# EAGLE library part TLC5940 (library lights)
16-channel LED Driver with Dot Correction and Grayscale PWM Control The TLC5940 is a 16-channel, constant-current sink LED driver. Each channel has an individually adjustable 4096-step grayscale PWM brightness control and a 64-step, constant-current sink (dot correction). The dot correction adjusts the brightness variations between LED channels and other LED drivers. The dot correction data is stored in an integrated EEPROM. Both grayscale control and dot correction are accessible via a serial interface. A single external resistor sets the maximum current value of all 16 channels. Packages: 28-pin HTSSOP 32-pin 5x5mm QFN 28-pin DIP
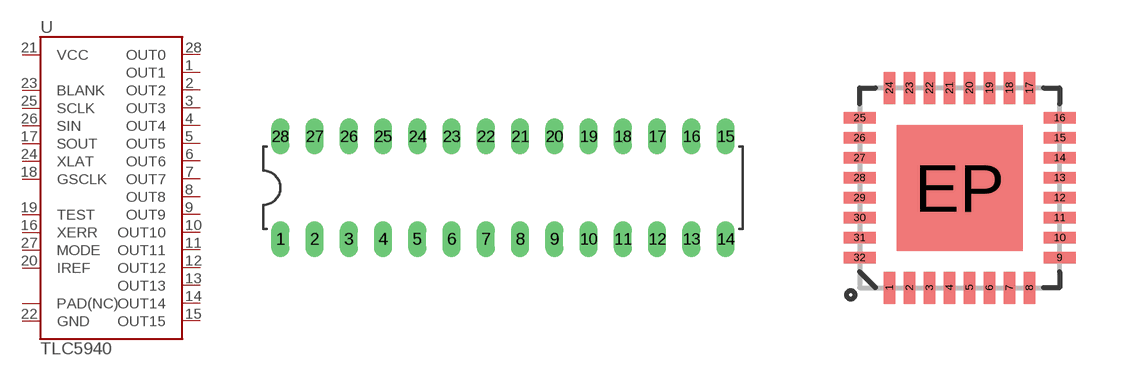
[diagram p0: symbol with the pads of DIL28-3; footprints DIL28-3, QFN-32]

Designator prefix U

## TLC5940-NT  [DIL28-3]
1  OUT1
2  OUT2
3  OUT3
4  OUT4
5  OUT5
6  OUT6
7  OUT7
8  OUT8
9  OUT9
10  OUT10
11  OUT11
12  OUT12
13  OUT13
14  OUT14
15  OUT15
16  XERR
17  SOUT
18  GSCLK
19  TEST
20  IREF
21  VCC
22  GND
23  BLANK
24  XLAT
25  SCLK
26  SIN
27  MODE
28  OUT0

## TLC5940-RHB (PROD_ID: IC-10398)  [QFN-32]
1  SCLK
2  SIN
3  MODE
4  OUT0
5  OUT1
6  OUT2
7  OUT3
8  OUT4
9  OUT5
10  OUT6
11  OUT7
14  OUT8
15  OUT9
16  OUT10
17  OUT11
18  OUT12
19  OUT13
20  OUT14
21  OUT15
22  XERR
23  SOUT
24  GSCLK
25  TEST
26  IREF
27  VCC
30  GND
31  BLANK
32  XLAT
EP  PAD(NC)

## TLC5940PWP  [TSSOP28-GROUNDPAD]
1  GND
2  BLANK
3  XLAT
4  SCLK
5  SIN
6  MODE
7  OUT0
8  OUT1
9  OUT2
10  OUT3
11  OUT4
12  OUT5
13  OUT6
14  OUT7
15  OUT8
16  OUT9
17  OUT10
18  OUT11
19  OUT12
20  OUT13
21  OUT14
22  OUT15
23  XERR
24  SOUT
25  GSCLK
26  TEST
27  IREF
28  VCC
29  PAD(NC)

## Footprint DIL28-3 (pad centres in mm)
Standard 28-pin DIP package. IC needs to have legs bent before insertion.
drill 0.813 long: 1 -16.51,-3.81; 2 -13.97,-3.81; 3 -11.43,-3.81; 4 -8.89,-3.81; 5 -6.35,-3.81; 6 -3.81,-3.81; 7 -1.27,-3.81; 8 1.27,-3.81; 9 3.81,-3.81; 10 6.35,-3.81; 11 8.89,-3.81; 12 11.43,-3.81; 13 13.97,-3.81; 14 16.51,-3.81; 15 16.51,3.81; 16 13.97,3.81; 17 11.43,3.81; 18 8.89,3.81; 19 6.35,3.81; 20 3.81,3.81; 21 1.27,3.81; 22 -1.27,3.81; 23 -3.81,3.81; 24 -6.35,3.81; 25 -8.89,3.81; 26 -11.43,3.81; 27 -13.97,3.81; 28 -16.51,3.81

## Footprint QFN-32 (pad centres in mm)
QFN 32-Pin package w/ Thermal Pad ***Unproven*** Applicable Parts: TLC5940
smd 0.285 x 0.8: 1 -1.75,-2.5; 2 -1.25,-2.5; 3 -0.75,-2.5; 4 -0.25,-2.5; 5 0.25,-2.5; 6 0.75,-2.5; 7 1.25,-2.5; 8 1.75,-2.5; 17 1.75,2.5; 18 1.25,2.5; 19 0.75,2.5; 20 0.25,2.5; 21 -0.25,2.5; 22 -0.75,2.5; 23 -1.25,2.5; 24 -1.75,2.5
smd 0.8 x 0.285: 9 2.5,-1.75; 10 2.5,-1.25; 11 2.5,-0.75; 12 2.5,-0.25; 13 2.5,0.25; 14 2.5,0.75; 15 2.5,1.25; 16 2.5,1.75; 25 -2.5,1.75; 26 -2.5,1.25; 27 -2.5,0.75; 28 -2.5,0.25; 29 -2.5,-0.25; 30 -2.5,-0.75; 31 -2.5,-1.25; 32 -2.5,-1.75
smd 3.15 x 3.15: EP 0,0

## Footprint TSSOP28-GROUNDPAD (pad centres in mm)
smd 0.8 x 0.25: 1 -2.921,4.298; 2 -2.921,3.637; 3 -2.921,2.977; 4 -2.921,2.317; 5 -2.921,1.656; 6 -2.921,0.996; 7 -2.921,0.335; 8 -2.927,-0.325; 9 -2.921,-0.985; 10 -2.921,-1.646; 11 -2.921,-2.306; 12 -2.921,-2.967; 13 -2.921,-3.627; 14 -2.921,-4.287; 15 2.921,-4.287; 16 2.921,-3.627; 17 2.921,-2.967; 18 2.921,-2.306; 19 2.921,-1.646; 20 2.921,-0.985; 21 2.927,-0.325; 22 2.921,0.335; 23 2.921,0.996; 24 2.921,1.656; 25 2.921,2.317; 26 2.921,2.977; 27 2.921,3.637; 28 2.921,4.298
smd 3.2 x 6.6: 29 0,0.005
